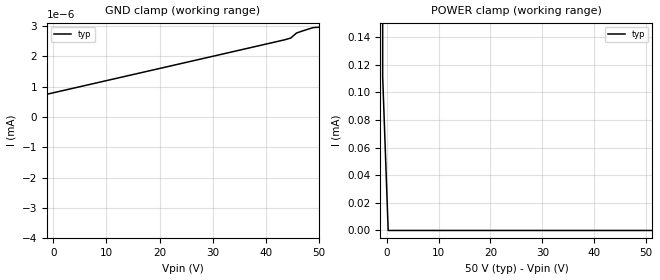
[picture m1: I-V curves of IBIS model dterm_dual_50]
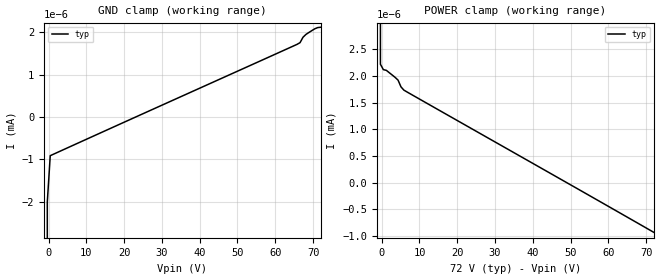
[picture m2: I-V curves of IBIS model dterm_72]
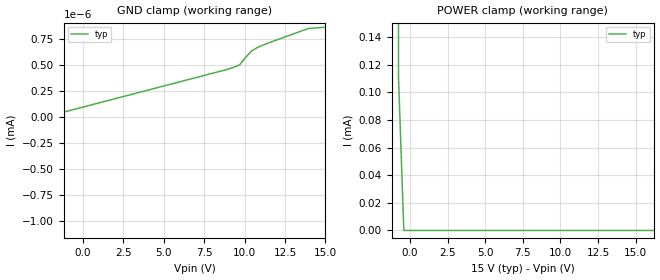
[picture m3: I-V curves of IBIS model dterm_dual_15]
|Texas Instruments Incorporated
|tmux8612, 4 Data Lane 1:1 220V Switch
[IBIS Ver]   4.1
[File name]   tmux8612.ibs
[Date]   02/11/25
[File Rev]   1.0
[Source]
| Texas Instruments Incorporated.
| ASC-INT-MPD
| 12500 TI Blvd
| Dallas, TX - 75243
[Notes]   Revision History:
| Rev 1.0: 02/11/25
| - Initial version of the model
| - Model generated from simulations in SPECTRE
| - C_comp although listed in numerical order of value are
|   obtained from varying PVT conditions. For PVT conditions for
|   each specific value refer the buffer description under
|   respective [Model]. IBIS model user is responsible for using
|   appropriate C_comp to simulate for Signal Integrity.
[Disclaimer]
| This model is designed as an aid for customers of Texas Instruments.
| TI and its licensors and suppliers make no warranties, either expressed
| or implied, with respect to this  model, including the warranties of
| merchantability or fitness for a particular purpose. The model is
| provided solely on an "as is" basis. The entire risk as to its quality
| and performance is with the customer.
| This model is subject to change without notice. Texas Instruments
| Incorporated is not responsible for updating this model.
[Copyright]
(C) Copyright 2025 Texas Instruments Incorporated.All rights reserved.
|  Component TMUX8612RUM 16-pin - RUM package
|  Part # TMUX8612RUM
[Component]   TMUX8612RUM
[Manufacturer]  TI
[Package]
|   typ   min   max
R_pkg   0.0668   NA   NA
L_pkg   2.1992nH   NA   NA
C_pkg   0.2884pF   NA   NA
[Pin]   signal_name   model_name
   1   VSS   power
   2   SEL1   inbuf
   3   GND   gnd
   4   SEL4   inbuf
   5   D4   dterm
   6   S4   sterm
   7   S3   sterm
   8   D3   dterm
   9   VDD   power
   10   NC   nc
   11   SEL3   inbuf
   12   SEL2   inbuf
   13   D2   dterm
   14   S2   sterm
   15   S1   sterm
   16   D1   dterm
[Series Switch Groups]
On 1 /
On 2 /
On 3 /
On 4 /
Off 1 /
[Series Pin Mapping]  pin_2 model_name function_table_group
  15  16   switch_dual_50   1
  14  13   switch_dual_50   1
   7   8   switch_dual_50   1
   6   5   switch_dual_50   1
|  15  16   switch_72   1
|  14  13   switch_72   1
|   7   8   switch_72   1
|   6   5   switch_72   1
|  15  16   switch_dual_15   1
|  14  13   switch_dual_15   1
|   7   8   switch_dual_15   1
|   6   5   switch_dual_15   1
|  15  16   switch_100   1
|  14  13   switch_100   1
|   7   8   switch_100   1
|   6   5   switch_100   1
|  15  16   switch_dual_36   1
|  14  13   switch_dual_36   1
|   7   8   switch_dual_36   1
|   6   5   switch_dual_36   1
[Model Selector] dterm
dterm_dual_50 Use for operation at +/-50V
dterm_72 Use for operation at 72V
dterm_dual_15 Use for operation at +/-15V
dterm_100 Use for operation at 100V
dterm_dual_36 Use for operation at +/-36V
[Model Selector] sterm
sterm_dual_50 Use for operation at +/-50V
sterm_72 Use for operation at 72V
sterm_dual_15 Use for operation at +/-15V
sterm_100 Use for operation at 100V
sterm_dual_36 Use for operation at +/-36V
[Model Selector] inbuf
inbuf_dual_50 Use for operation at +/-50V
inbuf_72 Use for operation at 72V
inbuf_dual_15 Use for operation at +/-15V
inbuf_100 Use for operation at 100V
inbuf_dual_36 Use for operation at +/-36V
| switch_dual_50
[Model]   switch_dual_50
Model_type   Series_switch
|   typ   min   max
C_comp   6.362683e-12   NA   NA
[Voltage Range]   50   NA   NA
[Power Clamp Reference]   50   NA   NA
[Temperature Range]   27   NA   NA
[On]
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[Off]
|   typ   min   max
[R Series]   10G   NA   NA
| switch_72
[Model]   switch_72
Model_type   Series_switch
|   typ   min   max
C_comp   1.008417e-11   NA   NA
[Voltage Range]   72   NA   NA
[Power Clamp Reference]   72   NA   NA
[Temperature Range]   27   NA   NA
[On]
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[Off]
|   typ   min   max
[R Series]   10G   NA   NA
| switch_dual_15
[Model]   switch_dual_15
Model_type   Series_switch
|   typ   min   max
C_comp   6.362683e-12   NA   NA
[Voltage Range]   15   NA   NA
[Power Clamp Reference]   15   NA   NA
[Temperature Range]   27   NA   NA
[On]
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[Off]
|   typ   min   max
[R Series]   10G   NA   NA
| switch_100
[Model]   switch_100
Model_type   Series_switch
|   typ   min   max
C_comp   1.008417e-11   NA   NA
[Voltage Range]   100   NA   NA
[Power Clamp Reference]   100   NA   NA
[Temperature Range]   27   NA   NA
[On]
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[Off]
|   typ   min   max
[R Series]   10G   NA   NA
| switch_dual_36
[Model]   switch_dual_36
Model_type   Series_switch
|   typ   min   max
C_comp   6.362683e-12   NA   NA
[Voltage Range]   36   NA   NA
[Power Clamp Reference]   36   NA   NA
[Temperature Range]   27   NA   NA
[On]
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[Off]
|   typ   min   max
[R Series]   10G   NA   NA
| Models and submodels in the file (20): dterm_dual_50 (Terminator), dterm_72 (Terminator), dterm_dual_15 (Terminator), dterm_100 (Terminator), dterm_dual_36 (Terminator), switch_dual_50 (Series_switch), switch_72 (Series_switch), switch_dual_15 (Series_switch), switch_100 (Series_switch), switch_dual_36 (Series_switch), sterm_dual_50 (Terminator), sterm_72 (Terminator), sterm_dual_15 (Terminator), sterm_100 (Terminator), sterm_dual_36 (Terminator), inbuf_dual_50 (Input), inbuf_72 (Input), inbuf_dual_15 (Input), inbuf_100 (Input), inbuf_dual_36 (Input)
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| dterm_dual_50
[Model]   dterm_dual_50
Model_type   Terminator
|   typ   min   max
C_comp   6.362683e-12   NA   NA
[Voltage Range]   50   NA   NA
[Temperature Range]   27   NA   NA
[Power Clamp Reference]   50   NA   NA
[GND Clamp Reference]   0   NA   NA
[GND Clamp]
|   Voltage   I(typ)   I(min)   I(max)
-55V      -2.409A    NA         NA
-50.76V   -1.565mA   NA         NA
-49.7V    -1.2nA     NA         NA
43.64V    2.55nA     NA         NA
44.7V     2.605nA    NA         NA
45.76V    2.767nA    NA         NA
48.94V    2.949nA    NA         NA
50V       2.96nA     NA         NA
[POWER Clamp]
|   Voltage   I(typ)   I(min)   I(max)
-5V       1.055A     NA         NA
-1.818V   191.2mA    NA         NA
-757.6mV  111.3uA    NA         NA
303mV     2.957nA    NA         NA
100V      -1.212nA   NA         NA
| dterm_72
[Model]   dterm_72
Model_type   Terminator
|   typ   min   max
C_comp   1.008417e-11   NA   NA
[Voltage Range]   72   NA   NA
[Temperature Range]   27   NA   NA
[Power Clamp Reference]   72   NA   NA
[GND Clamp Reference]   0   NA   NA
[GND Clamp]
|   Voltage   I(typ)   I(min)   I(max)
-5V       -2.409A    NA         NA
-1.111V   -48.12mA   NA         NA
-333.3mV  -2.008nA   NA         NA
444.4mV   -911.8pA   NA         NA
65.78V    1.717nA    NA         NA
66.56V    1.757nA    NA         NA
67.33V    1.884nA    NA         NA
68.11V    1.951nA    NA         NA
70.44V    2.083nA    NA         NA
72V       2.12nA     NA         NA
[POWER Clamp]
|   Voltage   I(typ)   I(min)   I(max)
-5V       1.055A     NA         NA
-1.111V   25.66mA    NA         NA
-333.3mV  2.216nA    NA         NA
444.4mV   2.116nA    NA         NA
1.222V    2.103nA    NA         NA
4.333V    1.919nA    NA         NA
5.111V    1.792nA    NA         NA
5.889V    1.731nA    NA         NA
72V       -929.9pA   NA         NA
| dterm_dual_15
[Model]   dterm_dual_15
Model_type   Terminator
|   typ   min   max
C_comp   6.362683e-12   NA   NA
[Voltage Range]   15   NA   NA
[Temperature Range]   27   NA   NA
[Power Clamp Reference]   15   NA   NA
[GND Clamp Reference]   0   NA   NA
[GND Clamp]
|   Voltage   I(typ)   I(min)   I(max)
-20V      -2.409A    NA         NA
-15.4V    -15.57nA   NA         NA
-15.05V   -514.1pA   NA         NA
8.99V     459.2pA    NA         NA
9.697V    500.3pA    NA         NA
10.4V     629.6pA    NA         NA
11.11V    687.7pA    NA         NA
13.94V    848.1pA    NA         NA
15V       860.4pA    NA         NA
[POWER Clamp]
|   Voltage   I(typ)   I(min)   I(max)
-5V       1.055A     NA         NA
-1.111V   25.67mA    NA         NA
-757.6mV  111.3uA    NA         NA
-404mV    1.902nA    NA         NA
30V       -512pA     NA         NA
